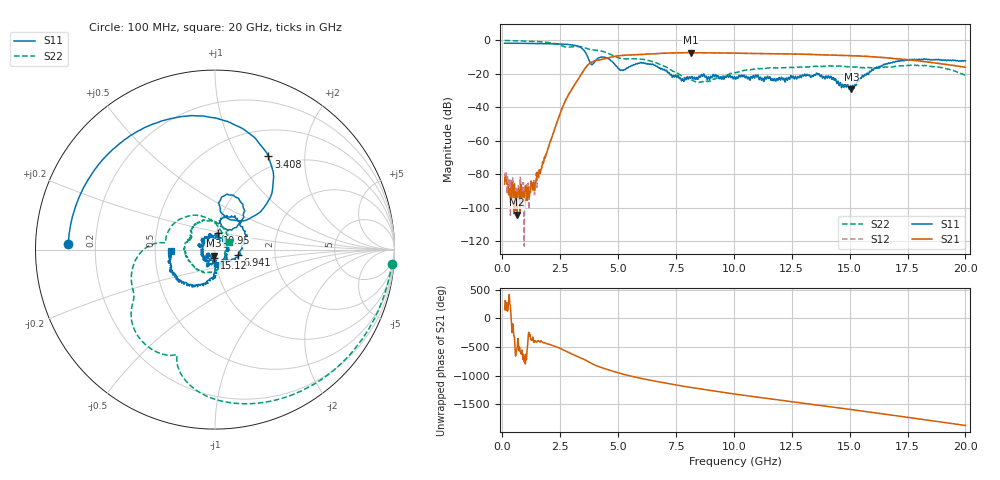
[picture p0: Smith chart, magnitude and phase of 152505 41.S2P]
!  2-Port S-parameters saved by WinCal
! VAR MeasName=S-Parameters (CALIBRATED_DATA) read from VNA (N5230C)
! VAR MeasDate=4/10/2015 9:32:34 AM
! VAR NAME=152505 41
! VAR FILENAME=152505 41.S2P
! VAR DATE=4/10/2015 9:32:34 AM
! VAR PHYS_PORTS=1,2
# Hz S DB R 50
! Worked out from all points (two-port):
!   801 points, 100 MHz to 20 GHz, reference 50 ohm
!   highest |S21| = -7.37 dB at 8.135 GHz (marker M1); lowest = -104.1 dB at 622.4 MHz (marker M2)
!   |S21| within 3 dB of the highest: 4.609 GHz to 16.5 GHz (11.89 GHz wide, 113 % of centre)
!   lowest |S11| = -29.2 dB at 15.07 GHz (marker M3), VSWR 1.07, Z = 49.3 - j3.36 ohm
!   |S11| at or under -10 dB: 3.692 GHz to 4.295 GHz (603.1 MHz wide, 15.1 % of centre); 4.359 GHz to end of sweep
!   |S22| runs from -25.3 to -0.1 dB; largest |S21 - S12| = 0.0067
!   S11 on the Smith chart (normalised r, x): 100 MHz: 0.10, +0.02; 3.408 GHz: 0.84, +1.36; 6.941 GHz: 1.29, -0.08; 10.95 GHz: 1.01, +0.19; 15.12 GHz: 0.98, -0.09; 20 GHz: 0.61, -0.01
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1e8  -1.75 177.6  -86.02 151.1  -82.35 0.4  -0.09 -4.6
6.22375e8  -1.78 165.1  -104.13 161.1  -87.82 -168.8  -0.30 -25.3
1.617375e9  -1.93 140.1  -78.16 -52.0  -78.03 -52.2  -0.84 -66.1
2.63725e9  -2.31 106.7  -38.73 167.4  -38.84 167.3  -3.69 -109.0
3.408375e9  -4.46 60.2  -20.26 25.6  -20.28 26.0  -3.87 -133.1
3.43325e9  -4.73 58.2  -19.72 21.2  -19.72 21.5  -3.93 -134.4
3.856125e9  -14.57 62.8  -13.02 -68.6  -13.06 -68.4  -5.65 -149.9
4.701875e9  -12.28 49.0  -10.07 164.1  -10.06 164.4  -8.55 177.3
5.497875e9  -15.75 81.7  -8.74 74.6  -8.74 74.4  -11.05 168.5
6.741625e9  -16.43 7.1  -7.86 -29.5  -7.86 -29.6  -13.96 111.5
6.940625e9  -17.68 -13.1  -7.72 -44.6  -7.72 -44.5  -15.19 101.1
8.134625e9  -22.70 -154.8  -7.37 -128.4  -7.38 -128.4  -23.51 38.8
9.055e9  -22.40 140.6  -7.50 173.9  -7.49 174.0  -23.82 -23.7
1.005e10  -22.11 126.5  -7.64 115.9  -7.68 115.7  -19.31 -79.3
1.09455e10  -20.66 80.2  -7.91 66.4  -7.86 66.7  -16.95 -114.1
1.218925e10  -24.15 -5.5  -8.14 -0.1  -8.12 -0.3  -16.40 -147.6
1.338325e10  -21.18 -102.1  -8.50 -64.3  -8.44 -64.0  -15.63 -166.1
1.507475e10  -29.20 -100.4  -9.22 -155.4  -9.20 -154.8  -15.96 161.4
1.51245e10  -26.83 -97.4  -9.25 -157.8  -9.25 -157.8  -15.96 161.7
1.669162e10  -13.48 -107.7  -10.58 114.5  -10.49 113.9  -16.07 148.3
1.83085e10  -11.18 -156.0  -12.89 24.3  -12.67 23.5  -15.10 110.6
2e10  -12.31 -178.6  -16.13 -72.6  -16.16 -72.6  -21.23 29.0
